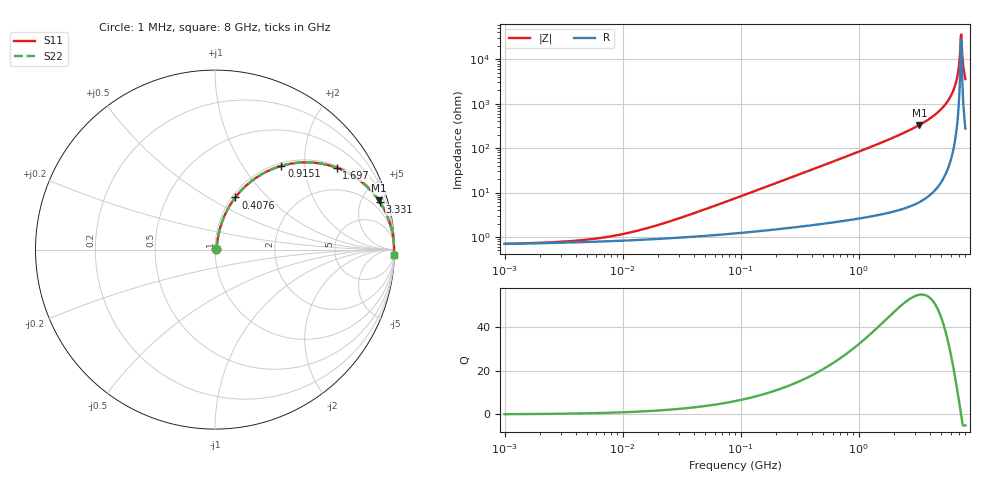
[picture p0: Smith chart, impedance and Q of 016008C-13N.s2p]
# MHz S MA R 50
!Freq  MagS11  AngS11  MagS21  AngS21  MagS12  AngS12  MagS22  AngS22
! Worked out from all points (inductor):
!   801 points, 1 MHz to 8 GHz, reference 50 ohm
!   read as one part in series: L = 13 nH near 36.82 MHz
!   highest Q = 54.5 at 3.257 GHz (marker M1), where L = 16.2 nH
!   self-resonance near 7.312 GHz
!   S11 on the Smith chart (normalised r, x): 1 MHz: 1.01, +0.00; 407.6 MHz: 1.04, +0.67; 915.1 MHz: 1.05, +1.52; 1.697 GHz: 1.07, +2.93; 3.331 GHz: 1.13, +6.84; 8 GHz: 6, -71
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1  0.006996 6.6  0.9931 -0.0  0.9931 -0.0  0.006996 6.6
4.505755  0.00844 25.4  0.9924 -0.2  0.9924 -0.2  0.00844 25.4
9.457416  0.0112 42.7  0.9918 -0.4  0.9918 -0.4  0.0112 42.7
20.07503  0.01857 60.1  0.9909 -0.9  0.9909 -0.9  0.01857 60.1
90.45318  0.07379 76.5  0.9854 -4.2  0.9854 -4.2  0.07379 76.5
198.584  0.1586 75.7  0.973 -9.1  0.973 -9.1  0.1586 75.7
403.007  0.3089 68.8  0.934 -18.0  0.934 -18.0  0.3089 68.8
407.5599  0.312 68.7  0.933 -18.2  0.933 -18.2  0.312 68.7
915.102  0.5955 51.6  0.784 -36.5  0.784 -36.5  0.5955 51.6
1697.489  0.8171 33.9  0.5578 -54.8  0.5578 -54.8  0.8171 33.9
1795.566  0.8334 32.3  0.5343 -56.4  0.5343 -56.4  0.8334 32.3
3256.724  0.9524 16.7  0.2878 -72.2  0.2878 -72.2  0.9524 16.7
3330.725  0.9552 16.2  0.2791 -72.7  0.2791 -72.7  0.9552 16.2
4718.277  0.9854 8.7  0.1505 -80.1  0.1505 -80.1  0.9854 8.7
5906.915  0.9948 4.2  0.07329 -83.9  0.07329 -83.9  0.9948 4.2
6609.207  0.9971 2.0  0.0357 -84.3  0.0357 -84.3  0.9971 2.0
6835.746  0.9975 1.4  0.02451 -83.4  0.02451 -83.4  0.9975 1.4
7149.923  0.9978 0.5  0.009721 -76.4  0.009721 -76.4  0.9978 0.5
7312.386  0.9978 0.1  0.002963 -42.6  0.002963 -42.6  0.9978 0.1
7563.027  0.9978 -0.5  0.009434 76.2  0.009434 76.2  0.9978 -0.5
7822.26  0.9976 -1.2  0.0205 82.8  0.0205 82.8  0.9976 -1.2
8000  0.9975 -1.6  0.02794 84.0  0.02794 84.0  0.9975 -1.6
